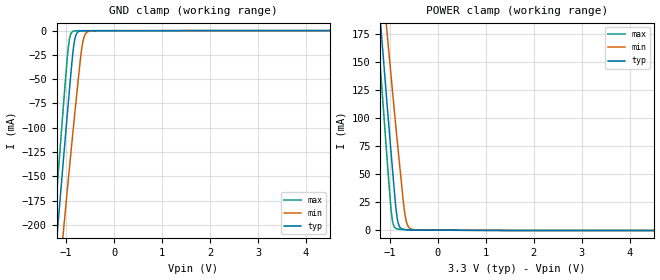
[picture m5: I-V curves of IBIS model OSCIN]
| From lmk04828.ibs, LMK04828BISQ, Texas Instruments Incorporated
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|   Model   OSCIN
[Model]   OSCIN
Model_type   Input
Vinl = 1.6
Vinh = 2.0
|   typ   min   max
|   (nom PVT)   (slow PVT)   (fast PVT)
C_comp   1.564pF   1.354pF   1.588pF
|C_comp (XTAL off)   1.564pF   1.354pF   1.588pF
|C_comp (XTAL on)   2.254pF   2.212pF   2.426pF
[Voltage Range]   3.3   3.15   3.45
[Temperature Range]   27   125   -40
[Power Clamp Reference]   3.3   3.15   3.45
[GND Clamp Reference]   0   0   0
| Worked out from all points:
|   GND clamp passes 1 mA (typ) near -0.74 V on its own axis
|   POWER clamp passes 1 mA (typ) near -0.71 V on its own axis
[GND Clamp]
|   Voltage   I(typ)   I(min)   I(max)
-3.3V     -1.495A    -1.435A    -1.554A
-1.261V   -253.6mA   -315.7mA   -208.6mA
-1.082V   -148mA     -220.4mA   -93.93mA
-1.053V   -130.6mA   -204.7mA   -75.15mA
-963.6mV  -79.45mA   -158.2mA   -21.35mA
-933.9mV  -62.73mA   -142.9mA   -9.671mA
-854.7mV  -20.63mA   -102.8mA   -658.8uA
-785.4mV  -3.401mA   -68.83mA   -184.8uA
-666.6mV  -218.4uA   -15.89mA   -123.8uA
-607.2mV  -143.9uA   -4.318mA   -121uA
-528mV    -125.7uA   -636.7uA   -120.6uA
6.6V      0A         0A         0A
[POWER Clamp]
|   Voltage   I(typ)   I(min)   I(max)
-3.3V     1.339A     1.265A     1.41A
-1.3V     241.3mA    290.6mA    205.4mA
-1.221V   198.6mA    252.8mA    158.6mA
-1.201V   188mA      243.4mA    146.9mA
-1.063V   114.5mA    177.9mA    66.18mA
-973.5mV  68.48mA    136.7mA    17.44mA
-933.9mV  48.52mA    118.6mA    5.959mA
-874.5mV  19.91mA    92.01mA    1.777mA
-805.2mV  3.93mA     61.83mA    1.123mA
-686.4mV  875.1uA    14.43mA    629.4uA
-537.9mV  429.7uA    1.008mA    382.6uA
6.6V      0A         0A         0A
